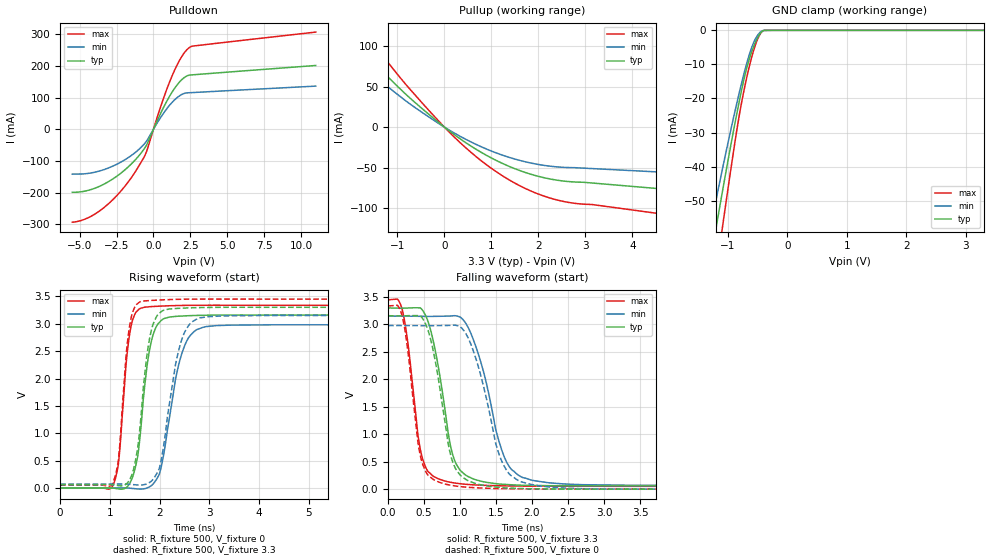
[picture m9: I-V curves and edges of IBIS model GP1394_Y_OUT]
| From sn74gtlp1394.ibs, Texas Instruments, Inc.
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[Model]   GP1394_Y_OUT
Model_type  3-state
Enable   Active-Low
Vref =   0.0
Rref =   500
Cref =   50p
Vmeas =   1.5
| variable   typ   min   max
C_comp   3.83pF   3.33pF   4.89pF
| C_pullup   4.35pF   3.69pF   5.29pF
| C_pulldown   5.95pF   3.50pF   7.85pF
| C_tri-state   3.83pF   3.33pF   4.89pF
[Temperature Range]   40   100   -40
| Ambient temperature   25   85   -40
[Voltage range]   3.3   3.15   3.45
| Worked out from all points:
|   slope of the pulldown table from 0 to 0.495 V, typ, clamps not added: 9.68 ohm
|   slope of the pullup table from 0 to 0.495 V, typ, clamps not added: 23.9 ohm
|   GND clamp passes 1 mA (typ) near -0.46 V on its own axis
|   rising waveform, R_fixture 500, V_fixture 0: 20-80 % time 232ps typ, 344ps min, 179ps max; typ from 0 V to 3.16 V
|   falling waveform, R_fixture 500, V_fixture 3.3: 20-80 % time 246ps typ, 350ps min, 183ps max; typ from 3.3 V to 0.06 V
|   rising waveform, R_fixture 500, V_fixture 3.3: 20-80 % time 228ps typ, 323ps min, 174ps max; typ from 0.06 V to 3.3 V
|   falling waveform, R_fixture 500, V_fixture 0: 20-80 % time 241ps typ, 335ps min, 180ps max; typ from 3.16 V to 0 V
[GND Clamp]
| GP1394_Y_OUT
|   Voltage   I(typ)   I(min)   I(max)
-5.5V     -552.1mA   -468.7mA   -683.7mA
-1.325V   -70.94mA   -60.7mA    -87.19mA
-1.27V    -65.27mA   -55.9mA    -80.16mA
-1.22V    -60.17mA   -51.58mA   -73.83mA
-1.165V   -54.61mA   -46.88mA   -66.92mA
-1.115V   -49.62mA   -42.65mA   -60.71mA
-1.065V   -44.69mA   -38.49mA   -54.57mA
-840mV    -23.57mA   -20.64mA   -28.22mA
-700mV    -12.21mA   -10.77mA   -15.18mA
-545mV    -3.831mA   -2.777mA   -4.688mA
-415mV    -209.3uA   -100.1uA   -188.6uA
3.3V      314pA      27.39nA    -8.968nA
[Pulldown]
| GP1394_Y_OUT
|   Voltage   I(typ)   I(min)   I(max)
-5.5V     -198.8mA   -141.6mA   -293.1mA
-4.5V     -193.6mA   -139.6mA   -280.6mA
-3.44V    -175.1mA   -128.5mA   -250.2mA
-2.36V    -143.8mA   -107.3mA   -202.9mA
-1.36V    -102.7mA   -77.8mA    -143.1mA
-490mV    -51.49mA   -38.59mA   -72.61mA
570mV     58.36mA    42.99mA    82.68mA
1.335V    122.5mA    88.34mA    176.3mA
1.895V    155.5mA    109.2mA    227.8mA
2.395V    170.5mA    115.2mA    256.4mA
2.68V     171.9mA    115.9mA    262.7mA
11V       201.3mA    136.2mA    306.7mA
[Pullup]
| GP1394_Y_OUT
|   Voltage   I(typ)   I(min)   I(max)
-5.5V     320.1mA    247.6mA    418.6mA
-2.805V   158.6mA    127.5mA    204.4mA
-2.315V   128.6mA    103.5mA    165.7mA
-2.18V    120.4mA    96.84mA    155mA
-1.86V    100.9mA    81.19mA    130.1mA
-1.675V   89.83mA    72.21mA    115.8mA
-680mV    33.11mA    26.37mA    43.26mA
550mV     -22.81mA   -17.82mA   -30.32mA
1.495V    -51.16mA   -39.3mA    -68.91mA
2.405V    -65.48mA   -49.06mA   -89.94mA
7.1V      -88.34mA   -62.9mA    -126.6mA
11V       -107.7mA   -74.59mA   -157.7mA
[Ramp]
| GP1394_Y_OUT
| variable   typ   min   max
dV/dt_r   1.91/2.37E-10   1.80/3.73E-10   2.02/1.91E-10
dV/dt_f   1.95/2.50E-10   1.85/3.63E-10   2.05/1.95E-10
R_load = 500
[Rising Waveform]
| GP1394_Y_OUT
R_fixture =   500
C_fixture =   0
L_fixture =   0
V_fixture =   0
V_fixture_min = 0
V_fixture_max = 0
|   Time   V(typ)   V(min)   V(max)
0s        -55.31nV   -121.7nV   135.5nV
1.065ns   -1.248mV   870.2uV    52.21mV
1.175ns   -16.5mV    1.904mV    463.7mV
1.415ns   109.5mV    -4.628mV   2.897V
1.565ns   602.3mV    -17.07mV   3.247V
1.715ns   1.967V     -9.473mV   3.305V
1.98ns    3.01V      222.6mV    3.321V
2.45ns    3.141V     2.459V     3.335V
2.94ns    3.156V     2.949V     3.339V
24.99ns   3.159V     2.979V     3.337V
[Falling Waveform]
| GP1394_Y_OUT
R_fixture =   500
C_fixture =   0
L_fixture =   0
V_fixture =   3.3
V_fixture_min = 3.15
V_fixture_max = 3.45
|   Time   V(typ)   V(min)   V(max)
0s        3.299V     3.15V      3.447V
205ps     3.296V     3.149V     3.224V
420ps     3.302V     3.148V     939.8mV
530ps     3.137V     3.146V     375.9mV
875ps     743mV      3.154V     123.8mV
1.035ns   303.5mV    3.096V     94.47mV
1.265ns   154.6mV    2.415V     73.11mV
1.65ns    85.19mV    484.1mV    59.51mV
2.23ns    63.18mV    116.5mV    54.02mV
24.99ns   59.84mV    71.41mV    50.36mV
[Rising Waveform]
| GP1394_Y_OUT
R_fixture =   500
C_fixture =   0
L_fixture =   0
V_fixture =   3.3
V_fixture_min = 3.15
V_fixture_max = 3.45
|   Time   V(typ)   V(min)   V(max)
0s        59.82mV    71.32mV    50.35mV
1.065ns   58.32mV    72.14mV    106.1mV
1.17ns    44.37mV    73.02mV    493.3mV
1.41ns    170.7mV    66.82mV    3.022V
1.56ns    729.3mV    55.65mV    3.368V
1.695ns   2.014V     62.29mV    3.417V
1.97ns    3.17V      306.8mV    3.433V
2.435ns   3.284V     2.675V     3.448V
2.94ns    3.298V     3.126V     3.451V
24.99ns   3.3V       3.15V      3.45V
[Falling Waveform]
| GP1394_Y_OUT
R_fixture =   500
C_fixture =   0
L_fixture =   0
V_fixture =   0
V_fixture_min = 0
V_fixture_max = 0
|   Time   V(typ)   V(min)   V(max)
0s        3.158V     2.979V     3.335V
205ps     3.155V     2.979V     3.1V
485ps     3.098V     2.977V     438.5mV
635ps     2.473V     2.977V     171mV
865ps     643.6mV    2.982V     72.68mV
1.03ns    222.6mV    2.923V     43.01mV
1.24ns    93.62mV    2.293V     23.48mV
1.605ns   25.36mV    438.9mV    9.638mV
2.205ns   3.839mV    43.49mV    3.778mV
24.99ns   23.44uV    84.5uV     15.61uV
